(* Logix 5000 AddOnInstructionDefinition export Banner_Q5X_2000_Param_v4; software revision 33.00; part 3 of 3 *)
(* tags used below, declared in another part *)
   Q5X : Banner_Q5X_2000_v4;
   Port_Data : Banner_IOL_Port_v4;
   Port : DINT;
   Local_Control : DINT;
   Command_Being_Processed : BOOL;
   Update_Archive : BOOL;
   Index_Write_Inprocess : INT;
   Inprocess_Index : DINT;
(* Banner_Q5X_2000_Param_v4, continued *)

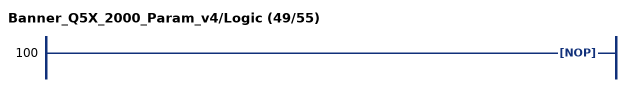
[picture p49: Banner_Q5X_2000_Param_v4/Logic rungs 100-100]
   100: NOP();
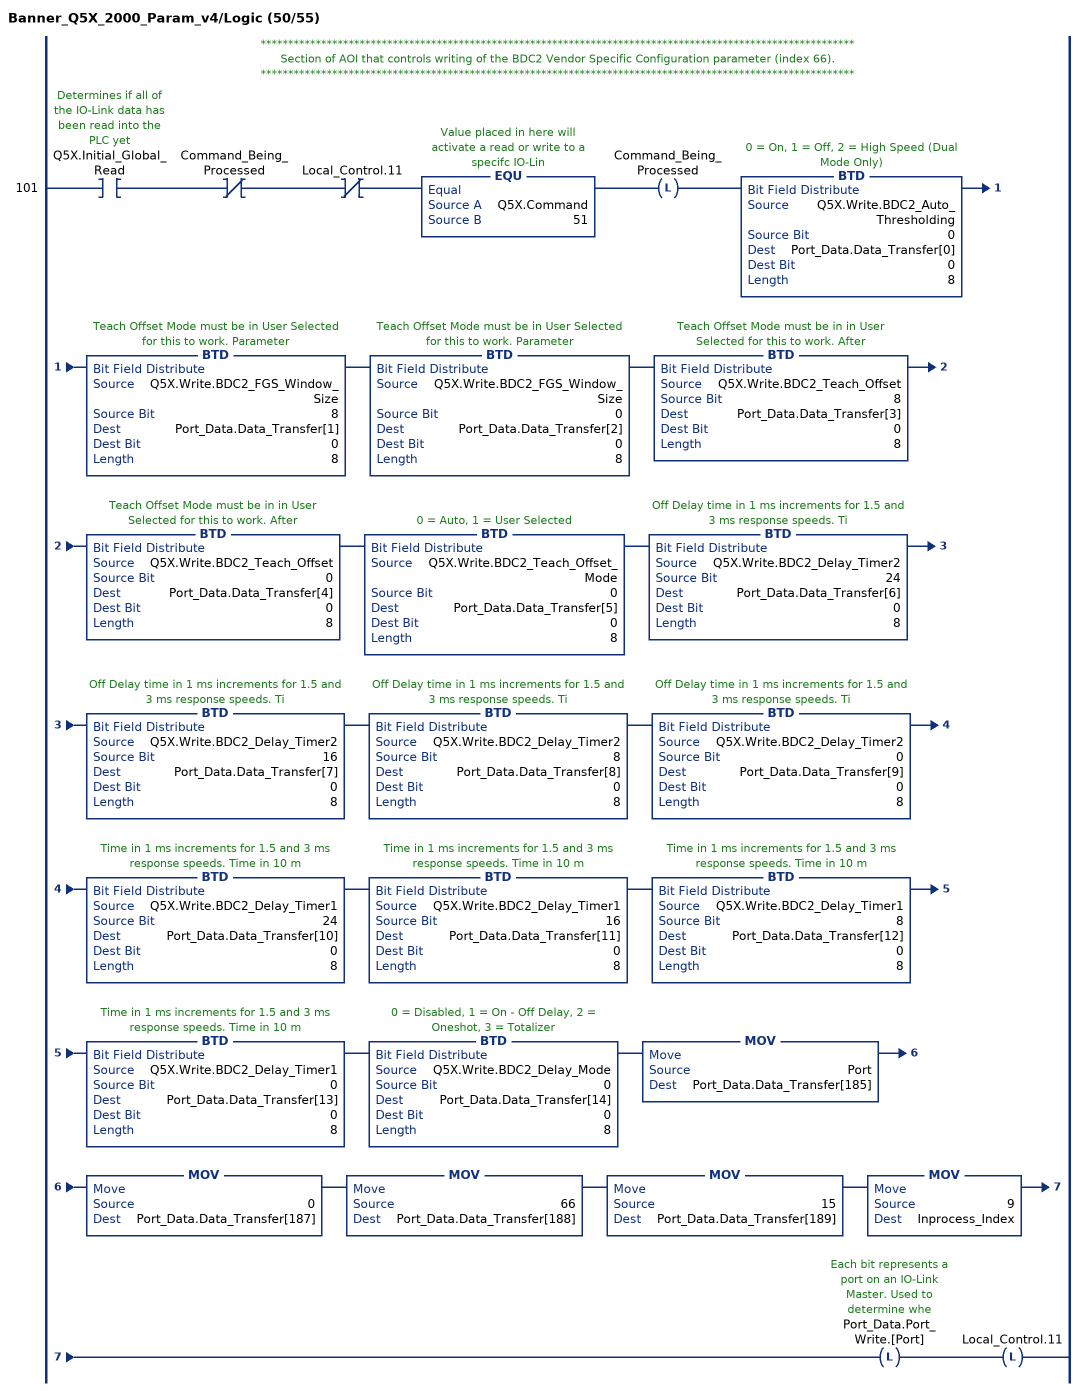
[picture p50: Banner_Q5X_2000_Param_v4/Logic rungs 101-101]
   // ************************************************************************************************************
   // Section of AOI that controls writing of the BDC2 Vendor Specific Configuration parameter (index 66).
   // ************************************************************************************************************
   101: XIC(Q5X.Initial_Global_Read)XIO(Command_Being_Processed)XIO(Local_Control.11)EQU(Q5X.Command,51)OTL(Command_Being_Processed)BTD(Q5X.Write.BDC2_Auto_Thresholding,0,Port_Data.Data_Transfer[0],0,8)BTD(Q5X.Write.BDC2_FGS_Window_Size,8,Port_Data.Data_Transfer[1],0,8)BTD(Q5X.Write.BDC2_FGS_Window_Size,0,Port_Data.Data_Transfer[2],0,8)BTD(Q5X.Write.BDC2_Teach_Offset,8,Port_Data.Data_Transfer[3],0,8)BTD(Q5X.Write.BDC2_Teach_Offset,0,Port_Data.Data_Transfer[4],0,8)BTD(Q5X.Write.BDC2_Teach_Offset_Mode,0,Port_Data.Data_Transfer[5],0,8)BTD(Q5X.Write.BDC2_Delay_Timer2,24,Port_Data.Data_Transfer[6],0,8)BTD(Q5X.Write.BDC2_Delay_Timer2,16,Port_Data.Data_Transfer[7],0,8)BTD(Q5X.Write.BDC2_Delay_Timer2,8,Port_Data.Data_Transfer[8],0,8)BTD(Q5X.Write.BDC2_Delay_Timer2,0,Port_Data.Data_Transfer[9],0,8)BTD(Q5X.Write.BDC2_Delay_Timer1,24,Port_Data.Data_Transfer[10],0,8)BTD(Q5X.Write.BDC2_Delay_Timer1,16,Port_Data.Data_Transfer[11],0,8)BTD(Q5X.Write.BDC2_Delay_Timer1,8,Port_Data.Data_Transfer[12],0,8)BTD(Q5X.Write.BDC2_Delay_Timer1,0,Port_Data.Data_Transfer[13],0,8)BTD(Q5X.Write.BDC2_Delay_Mode,0,Port_Data.Data_Transfer[14],0,8)MOV(Port,Port_Data.Data_Transfer[185])MOV(0,Port_Data.Data_Transfer[187])MOV(66,Port_Data.Data_Transfer[188])MOV(15,Port_Data.Data_Transfer[189])MOV(9,Inprocess_Index)OTL(Port_Data.Port_Write.[Port])OTL(Local_Control.11);
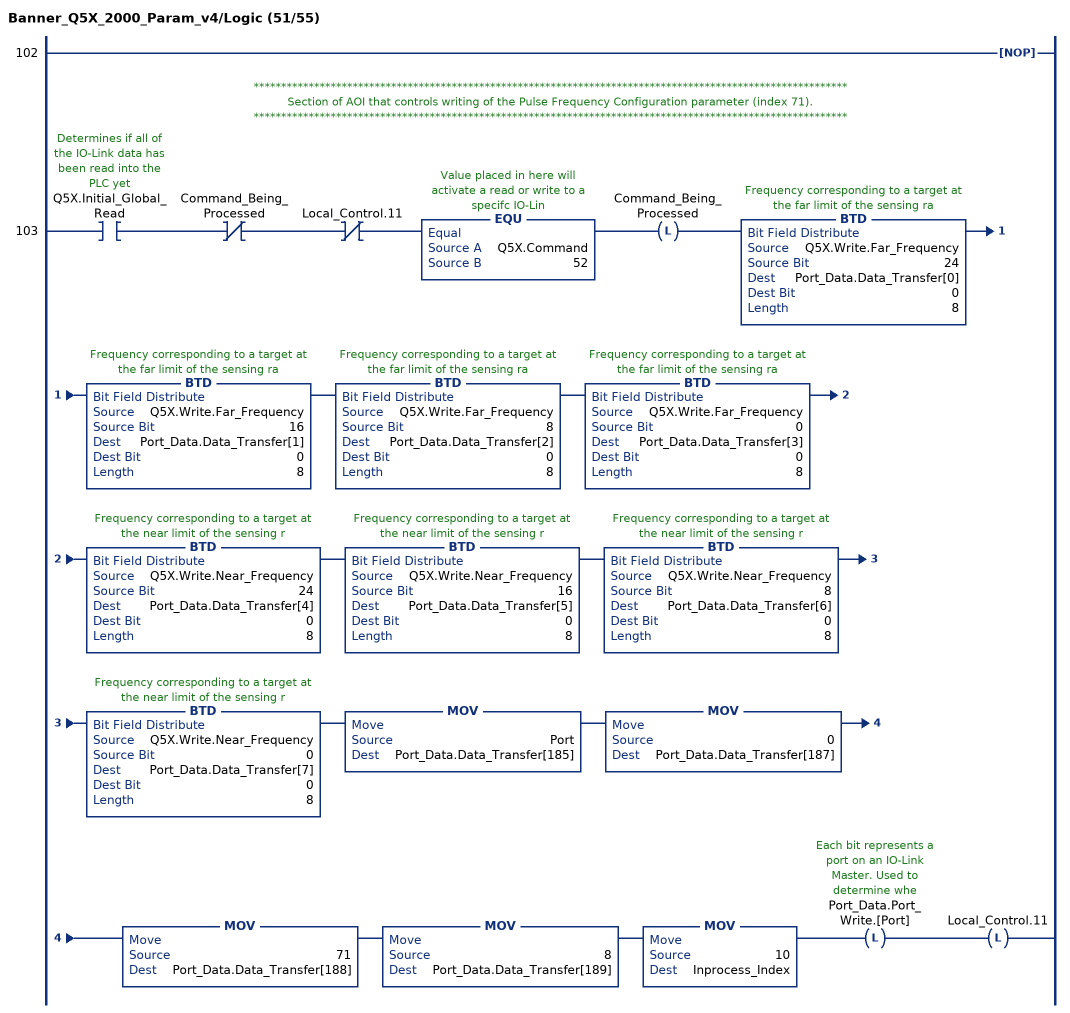
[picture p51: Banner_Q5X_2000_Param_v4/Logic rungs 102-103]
   102: NOP();
   // ************************************************************************************************************
   // Section of AOI that controls writing of the Pulse Frequency Configuration parameter (index 71).
   // ************************************************************************************************************
   103: XIC(Q5X.Initial_Global_Read)XIO(Command_Being_Processed)XIO(Local_Control.11)EQU(Q5X.Command,52)OTL(Command_Being_Processed)BTD(Q5X.Write.Far_Frequency,24,Port_Data.Data_Transfer[0],0,8)BTD(Q5X.Write.Far_Frequency,16,Port_Data.Data_Transfer[1],0,8)BTD(Q5X.Write.Far_Frequency,8,Port_Data.Data_Transfer[2],0,8)BTD(Q5X.Write.Far_Frequency,0,Port_Data.Data_Transfer[3],0,8)BTD(Q5X.Write.Near_Frequency,24,Port_Data.Data_Transfer[4],0,8)BTD(Q5X.Write.Near_Frequency,16,Port_Data.Data_Transfer[5],0,8)BTD(Q5X.Write.Near_Frequency,8,Port_Data.Data_Transfer[6],0,8)BTD(Q5X.Write.Near_Frequency,0,Port_Data.Data_Transfer[7],0,8)MOV(Port,Port_Data.Data_Transfer[185])MOV(0,Port_Data.Data_Transfer[187])MOV(71,Port_Data.Data_Transfer[188])MOV(8,Port_Data.Data_Transfer[189])MOV(10,Inprocess_Index)OTL(Port_Data.Port_Write.[Port])OTL(Local_Control.11);
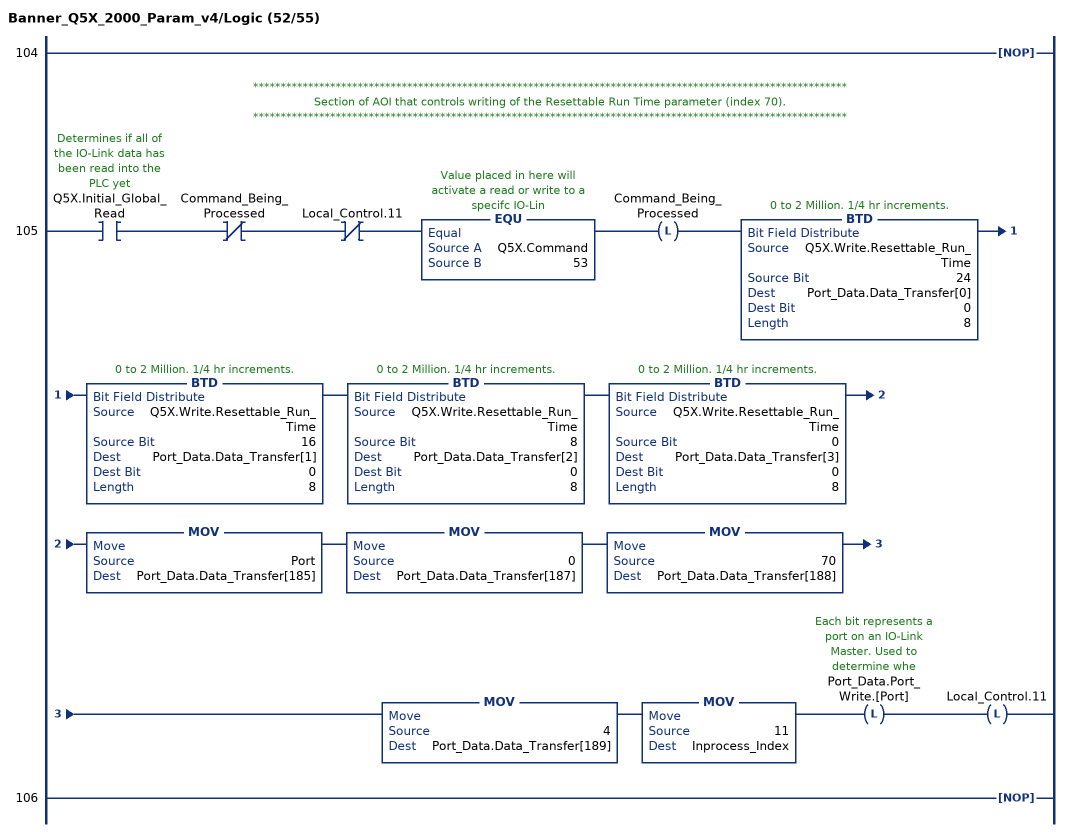
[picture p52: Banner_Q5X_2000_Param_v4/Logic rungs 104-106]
   104: NOP();
   // ************************************************************************************************************
   // Section of AOI that controls writing of the Resettable Run Time parameter (index 70).
   // ************************************************************************************************************
   105: XIC(Q5X.Initial_Global_Read)XIO(Command_Being_Processed)XIO(Local_Control.11)EQU(Q5X.Command,53)OTL(Command_Being_Processed)BTD(Q5X.Write.Resettable_Run_Time,24,Port_Data.Data_Transfer[0],0,8)BTD(Q5X.Write.Resettable_Run_Time,16,Port_Data.Data_Transfer[1],0,8)BTD(Q5X.Write.Resettable_Run_Time,8,Port_Data.Data_Transfer[2],0,8)BTD(Q5X.Write.Resettable_Run_Time,0,Port_Data.Data_Transfer[3],0,8)MOV(Port,Port_Data.Data_Transfer[185])MOV(0,Port_Data.Data_Transfer[187])MOV(70,Port_Data.Data_Transfer[188])MOV(4,Port_Data.Data_Transfer[189])MOV(11,Inprocess_Index)OTL(Port_Data.Port_Write.[Port])OTL(Local_Control.11);
   106: NOP();
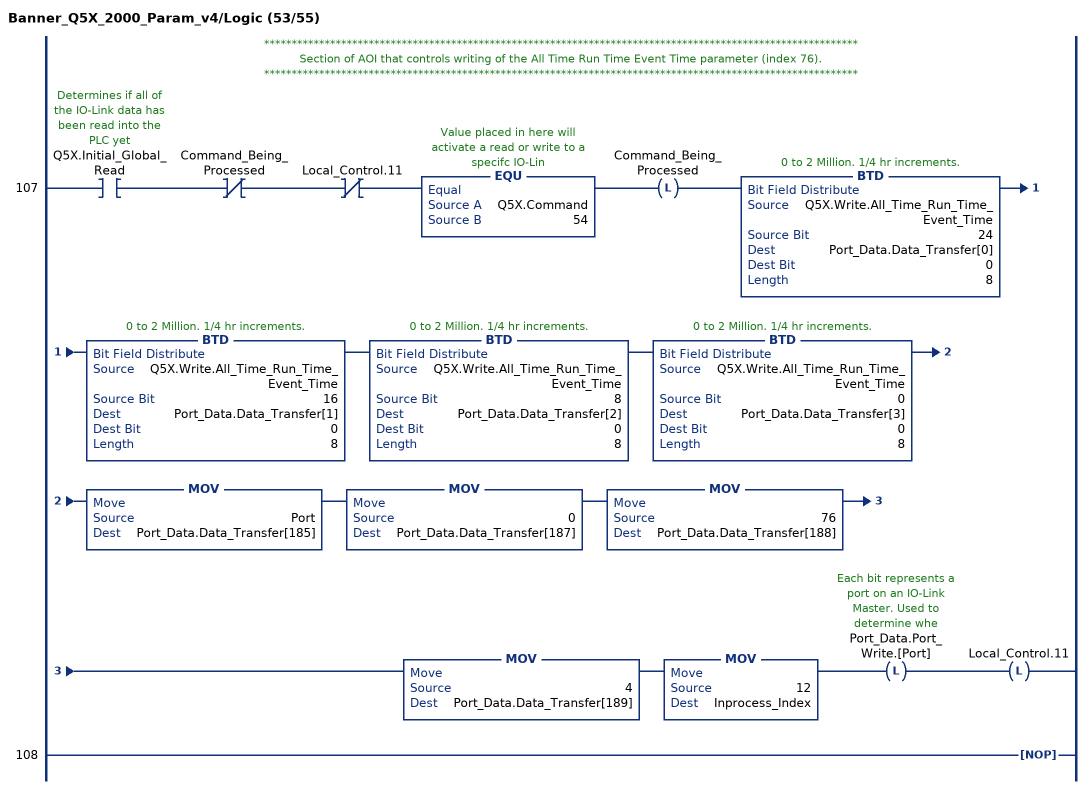
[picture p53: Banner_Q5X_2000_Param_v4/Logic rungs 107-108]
   // ************************************************************************************************************
   // Section of AOI that controls writing of the All Time Run Time Event Time parameter (index 76).
   // ************************************************************************************************************
   107: XIC(Q5X.Initial_Global_Read)XIO(Command_Being_Processed)XIO(Local_Control.11)EQU(Q5X.Command,54)OTL(Command_Being_Processed)BTD(Q5X.Write.All_Time_Run_Time_Event_Time,24,Port_Data.Data_Transfer[0],0,8)BTD(Q5X.Write.All_Time_Run_Time_Event_Time,16,Port_Data.Data_Transfer[1],0,8)BTD(Q5X.Write.All_Time_Run_Time_Event_Time,8,Port_Data.Data_Transfer[2],0,8)BTD(Q5X.Write.All_Time_Run_Time_Event_Time,0,Port_Data.Data_Transfer[3],0,8)MOV(Port,Port_Data.Data_Transfer[185])MOV(0,Port_Data.Data_Transfer[187])MOV(76,Port_Data.Data_Transfer[188])MOV(4,Port_Data.Data_Transfer[189])MOV(12,Inprocess_Index)OTL(Port_Data.Port_Write.[Port])OTL(Local_Control.11);
   108: NOP();
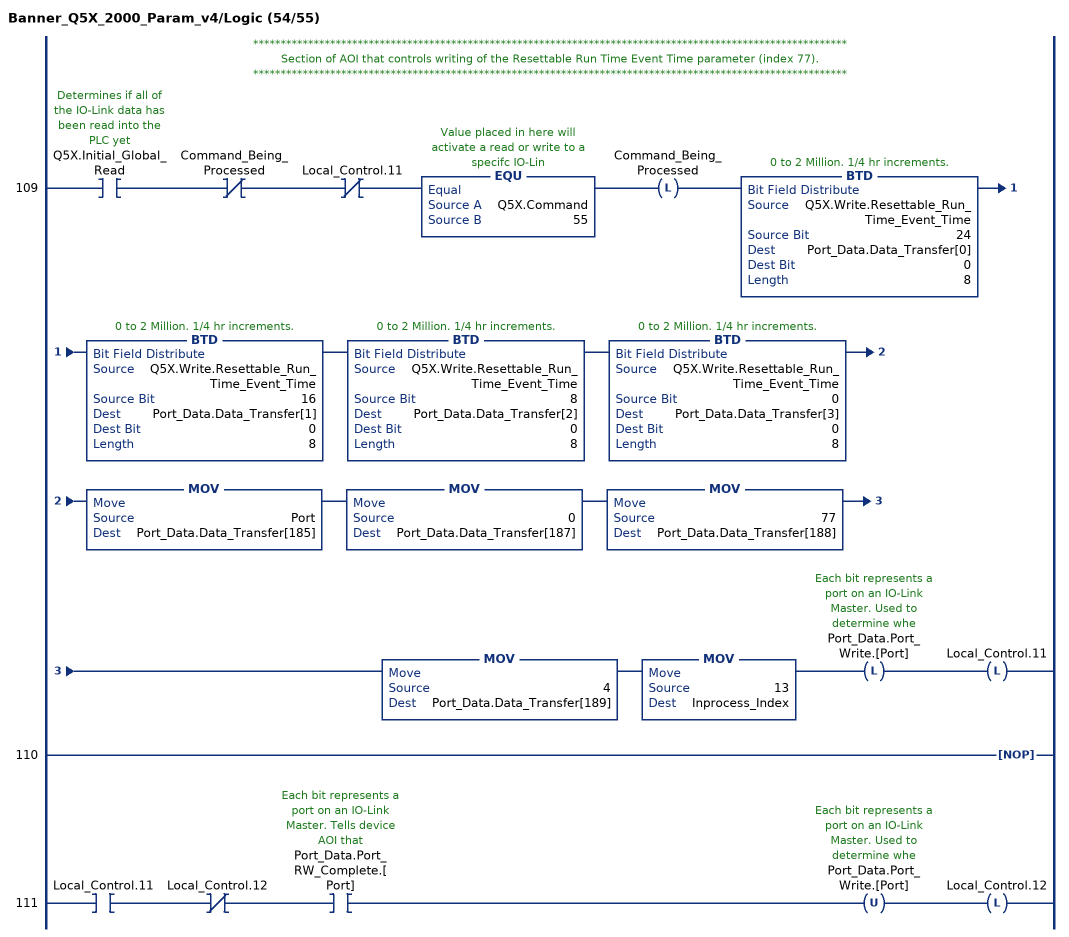
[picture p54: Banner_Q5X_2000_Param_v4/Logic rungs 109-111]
   // ************************************************************************************************************
   // Section of AOI that controls writing of the Resettable Run Time Event Time parameter (index 77).
   // ************************************************************************************************************
   109: XIC(Q5X.Initial_Global_Read)XIO(Command_Being_Processed)XIO(Local_Control.11)EQU(Q5X.Command,55)OTL(Command_Being_Processed)BTD(Q5X.Write.Resettable_Run_Time_Event_Time,24,Port_Data.Data_Transfer[0],0,8)BTD(Q5X.Write.Resettable_Run_Time_Event_Time,16,Port_Data.Data_Transfer[1],0,8)BTD(Q5X.Write.Resettable_Run_Time_Event_Time,8,Port_Data.Data_Transfer[2],0,8)BTD(Q5X.Write.Resettable_Run_Time_Event_Time,0,Port_Data.Data_Transfer[3],0,8)MOV(Port,Port_Data.Data_Transfer[185])MOV(0,Port_Data.Data_Transfer[187])MOV(77,Port_Data.Data_Transfer[188])MOV(4,Port_Data.Data_Transfer[189])MOV(13,Inprocess_Index)OTL(Port_Data.Port_Write.[Port])OTL(Local_Control.11);
   110: NOP();
   111: XIC(Local_Control.11)XIO(Local_Control.12)XIC(Port_Data.Port_RW_Complete.[Port])OTU(Port_Data.Port_Write.[Port])OTL(Local_Control.12);
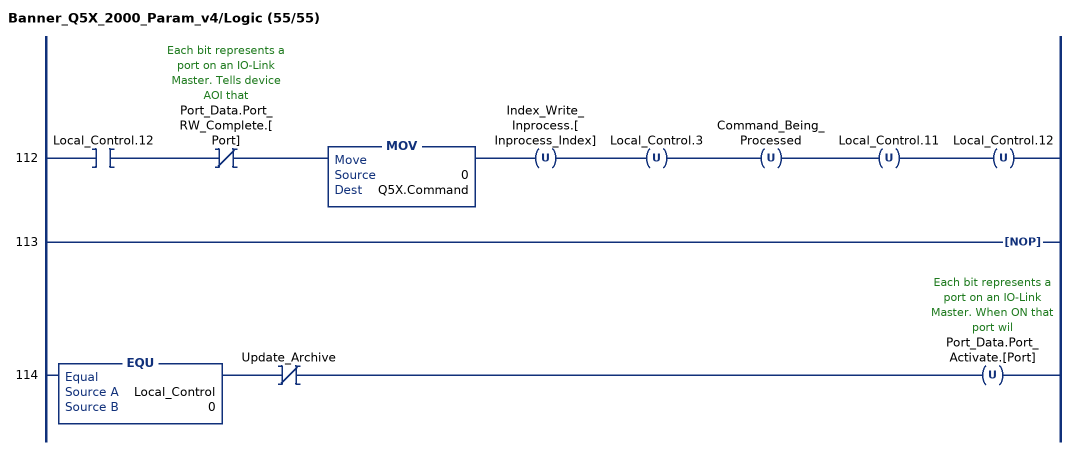
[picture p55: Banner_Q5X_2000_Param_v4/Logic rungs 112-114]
   112: XIC(Local_Control.12)XIO(Port_Data.Port_RW_Complete.[Port])MOV(0,Q5X.Command)OTU(Index_Write_Inprocess.[Inprocess_Index])OTU(Local_Control.3)OTU(Command_Being_Processed)OTU(Local_Control.11)OTU(Local_Control.12);
   113: NOP();
   114: EQU(Local_Control,0)XIO(Update_Archive)OTU(Port_Data.Port_Activate.[Port]);
END_ROUTINE
END_ADD_ON_INSTRUCTION
